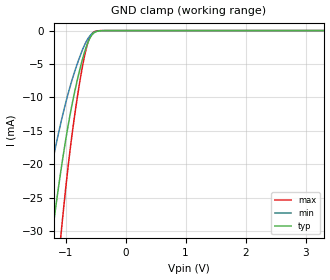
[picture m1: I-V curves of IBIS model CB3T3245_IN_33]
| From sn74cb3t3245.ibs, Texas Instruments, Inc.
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[Model]   CB3T3245_IN_33
Model_type  Input
Vinl=0.8
Vinh=2.0
| variable   typ   min   max
C_comp   2.65pF   1.99pF   3.02pF
[Temperature Range]   40   100   -40
| Ambient temperature   25   85   -40
[Voltage range]   3.3   3   3.6
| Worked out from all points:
|   GND clamp passes 1 mA (typ) near -0.59 V on its own axis
[GND Clamp]
| CB3T3245_IN_33
|   Voltage   I(typ)   I(min)   I(max)
-5V       -417.4mA   -313.8mA   -530.2mA
-1.44V    -46.78mA   -30.7mA    -68.45mA
-1.415V   -44.79mA   -29.37mA   -65.63mA
-1.215V   -29.92mA   -19.56mA   -44.07mA
-1.075V   -20.82mA   -13.68mA   -30.43mA
-915mV    -12.14mA   -8.092mA   -17.17mA
-775mV    -6.293mA   -4.223mA   -8.327mA
-705mV    -3.871mA   -2.604mA   -4.738mA
-640mV    -2.061mA   -1.399mA   -2.176mA
-585mV    -984.6uA   -696.2uA   -825.5uA
-530mV    -367.5uA   -288.3uA   -219.4uA
3.3V      128.8pA    501.8pA    26.94pA
